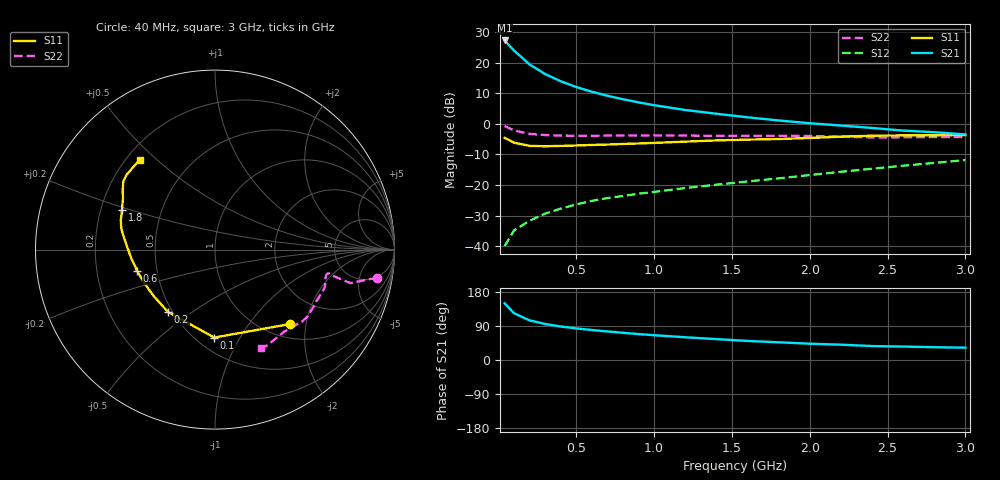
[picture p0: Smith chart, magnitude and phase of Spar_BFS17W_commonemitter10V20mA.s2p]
! Filename:  BFS17WJ.S2P  Version:  4.0
! NXP part #: BFS17W  Date: Jun 1994
! Bias condition: Vce=10V, Ic=20mA
#  MHz  S  MA  R  50
! Freq  S11  S21  S12  S22  !GUM [dB]
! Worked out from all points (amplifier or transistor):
!   21 points, 40 MHz to 3 GHz, reference 50 ohm
!   highest |S21| = 27.2 dB at 40 MHz (marker M1)
!   |S21| within 3 dB of that: start of sweep to 94.96 MHz
!   unconditionally stable (mu >= 1): 318.1 MHz to 2.248 GHz
!   at 300 MHz: K = 0.98, MSG = 22.8 dB, |S12| = -29.4 dB
!   at 1 GHz: K = 1.23, MAG = 11.3 dB, |S12| = -22.3 dB
!   at 3 GHz: K = 0.94, MSG = 4.2 dB, |S12| = -11.9 dB
!   S11 on the Smith chart (normalised r, x): 40 MHz: 1.28, -1.62; 100 MHz: 0.61, -0.78; 200 MHz: 0.47, -0.41; 600 MHz: 0.39, -0.11; 1.8 GHz: 0.29, +0.19; 3 GHz: 0.25, +0.44
40  0.588 -44.9  22.92 149.6  0.01 71.7  0.918 -9.8
100  0.49 -90.5  15.72 123.6  0.018 59.8  0.777 -13.9
200  0.435 -126.9  9.326 104.6  0.026 59.7  0.683 -12.7
300  0.429 -143.5  6.485 95.1  0.034 61.7  0.653 -11.8
400  0.434 -153.4  4.944 88.4  0.041 63.9  0.64 -12.1
500  0.441 -159.7  3.976 83.4  0.048 65.5  0.635 -13.1
600  0.45 -164.8  3.333 79.2  0.055 67.1  0.636 -14.3
700  0.457 -169.2  2.865 75.3  0.061 68.5  0.639 -15.6
800  0.467 -173.2  2.512 71.8  0.066 69.7  0.643 -17.0
900  0.476 -177.0  2.233 68.4  0.072 70.9  0.645 -18.2
1000  0.486 179.3  2.007 65.4  0.077 72.3  0.646 -19.6
1200  0.51 172.9  1.677 60.0  0.089 75.2  0.64 -22.8
1400  0.534 167.6  1.456 55.1  0.101 78.6  0.634 -27.0
1600  0.55 162.6  1.274 50.3  0.114 81.6  0.635 -31.7
1800  0.563 157.0  1.13 46.7  0.128 84.6  0.636 -35.6
2000  0.585 151.3  1.019 43.0  0.145 87.1  0.63 -39.3
2200  0.614 146.8  0.934 40.4  0.164 88.9  0.613 -43.9
2400  0.638 143.2  0.853 36.8  0.184 90.1  0.598 -49.8
2600  0.645 139.9  0.772 35.4  0.206 90.7  0.6 -56.0
2800  0.647 135.4  0.727 33.8  0.229 91.0  0.608 -60.9
3000  0.653 129.9  0.669 32.5  0.255 91.0  0.606 -64.7
